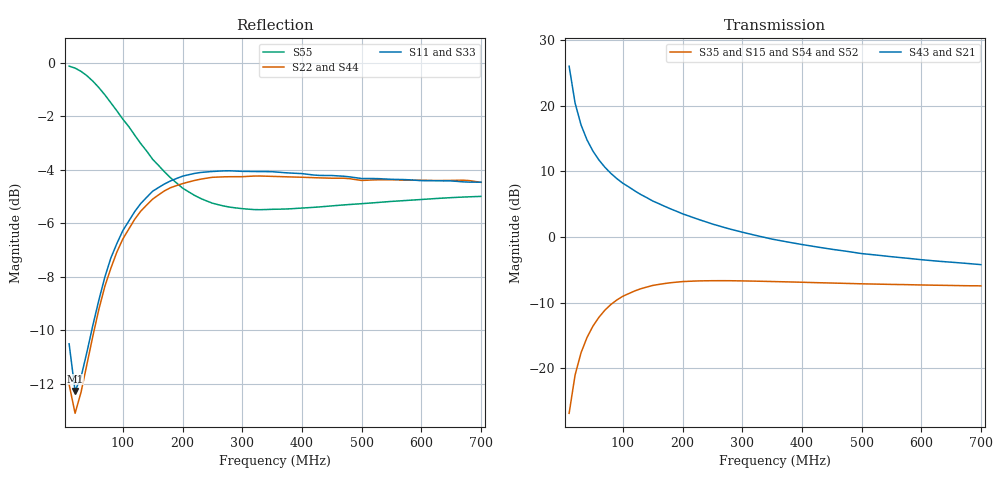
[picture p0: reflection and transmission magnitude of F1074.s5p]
! Date: Mon Aug 07 16:58:30 1995
!  POLYFET RF DEVICES
!  F1074 (Each Side)
!  S PARAMETERS
!  VDS=28V, IDQ=800mA
!AWR Design Environment (2053) Wed Feb 04 14:33:20 2004
!freq-unit  param-type  data-format  keyword  impedance-ohms
# MHz  S  MA  R  50
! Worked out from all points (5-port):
!   70 points, 10 MHz to 700 MHz, reference 50 ohm
!   strongest paths, dB at 10 MHz, 180 MHz, 360 MHz, 530 MHz, 700 MHz:
!     S43: 26.0, 4.3, -0.5, -2.8, -4.2
!     S21: 26.0, 4.3, -0.5, -2.8, -4.2
!     S35: -26.9, -7.0, -6.8, -7.2, -7.5
!     S15: -26.9, -7.0, -6.8, -7.2, -7.5
!     S54: -27.2, -7.2, -6.9, -7.2, -7.4
!     S52: -27.2, -7.2, -6.9, -7.2, -7.4
!   lowest |S11| = -12.3 dB at 20 MHz (marker M1), VSWR 1.64, Z = 49.1 - j24.8 ohm
!   |S11| at or under -10 dB: start of sweep to 47.96 MHz
